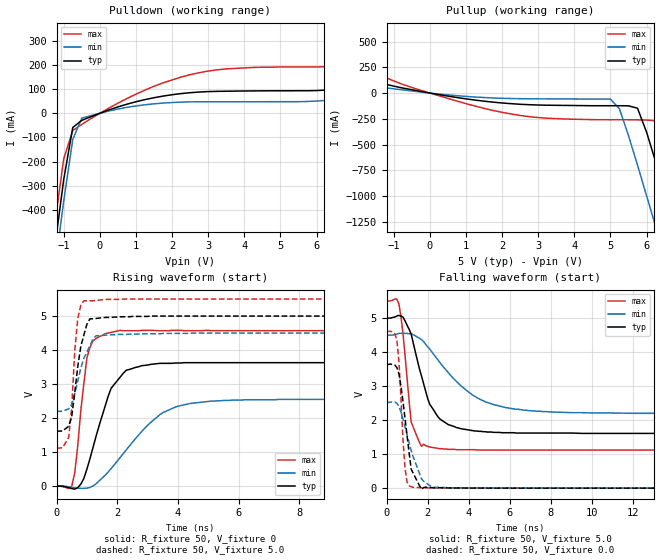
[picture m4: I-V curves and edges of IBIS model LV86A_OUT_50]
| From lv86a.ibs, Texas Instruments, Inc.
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|   Model LV86A_OUT_50
[Model]   LV86A_OUT_50
Model_type  Output
Polarity   Non-Inverting
Vmeas = 2.50v
Cref = 15pf
| variable   typ   min   max
C_comp   4.62pf   3.47pf   5.77pf
[Temperature Range]   25   85   -40
[Voltage Range]   5.0   4.5   5.5
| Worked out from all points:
|   slope of the pulldown table from 0 to 0.75 V, typ, clamps not added: 19.9 ohm
|   slope of the pullup table from 0 to 0.75 V, typ, clamps not added: 17.2 ohm
|   rising waveform, R_fixture 50, V_fixture 0: 20-80 % time 747ps typ, 1.54ns min, 320ps max; typ from 0 V to 3.63 V
|   falling waveform, R_fixture 50, V_fixture 5.0: 20-80 % time 1.02ns typ, 2.24ns min, 406ps max; typ from 5 V to 1.61 V
|   rising waveform, R_fixture 50, V_fixture 5.0: 20-80 % time 329ps typ, 472ps min, 203ps max; typ from 1.61 V to 5 V
|   falling waveform, R_fixture 50, V_fixture 0.0: 20-80 % time 442ps typ, 750ps min, 255ps max; typ from 3.64 V to 0 V
[Pulldown]
|   Voltage   I(typ)   I(min)   I(max)
-5V       -5.14A     -5.22A     -5.05A
-1.25V    -557mA     -649mA     -461mA
-1V       -274mA     -363mA     -188mA
-750mV    -58.9mA    -108mA     -71.3mA
-500mV    -29.2mA    -20mA      -46.2mA
0V        -3.33nA    -3.4nA     -3.57nA
1.25V     56.7mA     35.2mA     96mA
2.5V      85.3mA     47.3mA     160mA
3.5V      91.4mA     47.8mA     184mA
7V        108mA      63mA       206mA
8.25V     142mA      85.5mA     255mA
10V       202mA      122mA      357mA
[Pullup]
|   Voltage   I(typ)   I(min)   I(max)
-5V       343mA      194mA      632mA
-750mV    48.6mA     30.8mA     83.5mA
1.25V     -68.2mA    -38.5mA    -126mA
3V        -116mA     -56.1mA    -238mA
5V        -123mA     -58.9mA    -259mA
5.25V     -123mA     -153mA     -259mA
5.75V     -147mA     -699mA     -260mA
6.25V     -664mA     -1.29A     -268mA
6.5V      -960mA     -1.6A      -403mA
6.75V     -1.26A     -1.9A      -685mA
7.25V     -1.87A     -2.51A     -1.28A
10V       -5.25A     -5.89A     -4.66A
[Ramp]
| variable   typ   min   max
dV/dt_r   2.18E+00/7.67E-10   1.54E+00/1.53E-09   2.80E+00/3.06E-10
dV/dt_f   2.08E+00/9.83E-10   1.41E+00/2.26E-09   2.67E+00/4.25E-10
R_load = 50
[Rising Waveform]
R_fixture = 50
V_fixture = 0
|   Time   V(typ)   V(min)   V(max)
0s        0V         0V         0V
500ps     -71.8mV    -37.7mV    -7.09mV
600ps     -89.1mV    -50.9mV    388mV
1ns       500mV      -60.3mV    3.77V
1.1ns     804mV      -37.2mV    4.08V
1.7ns     2.64V      415mV      4.5V
2.1ns     3.21V      848mV      4.58V
3.5ns     3.61V      2.16V      4.57V
5.1ns     3.63V      2.5V       4.57V
25ns      3.63V      2.55V      4.57V
[Falling Waveform]
R_fixture = 50
V_fixture = 5.0
V_fixture_min = 4.5
V_fixture_max = 5.5
|   Time   V(typ)   V(min)   V(max)
0s        5V         4.5V       5.5V
600ps     5.08V      4.55V      5.42V
800ps     5.03V      4.56V      4.55V
1.2ns     4.53V      4.54V      1.94V
1.7ns     3.3V       4.37V      1.23V
2.1ns     2.47V      4.09V      1.21V
3ns       1.87V      3.4V       1.14V
4.4ns     1.68V      2.66V      1.12V
6.3ns     1.62V      2.32V      1.12V
25ns      1.61V      2.2V       1.12V
[Rising Waveform]
R_fixture = 50
V_fixture = 5.0
V_fixture_min = 4.5
V_fixture_max = 5.5
|   Time   V(typ)   V(min)   V(max)
0s        1.61V      2.2V       1.12V
400ps     1.76V      2.27V      1.43V
500ps     2.04V      2.41V      2.3V
600ps     2.74V      2.72V      3.98V
700ps     3.52V      3.09V      4.93V
900ps     4.44V      3.76V      5.45V
1.1ns     4.92V      4.13V      5.45V
1.3ns     4.93V      4.42V      5.46V
2ns       4.97V      4.46V      5.49V
25ns      5V         4.5V       5.5V
[Falling Waveform]
R_fixture = 50
V_fixture = 0.0
|   Time   V(typ)   V(min)   V(max)
0s        3.64V      2.53V      4.61V
500ps     3.55V      2.5V       4.37V
600ps     3.37V      2.41V      3.75V
900ps     2.05V      1.81V      595mV
1ns       1.54V      1.57V      171mV
1.2ns     556mV      1.1V       41.9mV
1.3ns     436mV      918mV      23.3mV
1.7ns     -30.2mV    275mV      12mV
2.3ns     12.3mV     23.1mV     4.86mV
25ns      0V         0V         5.8uV
